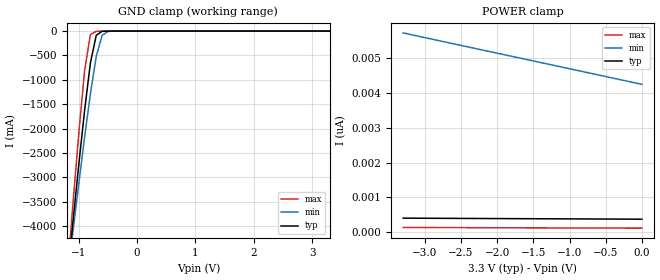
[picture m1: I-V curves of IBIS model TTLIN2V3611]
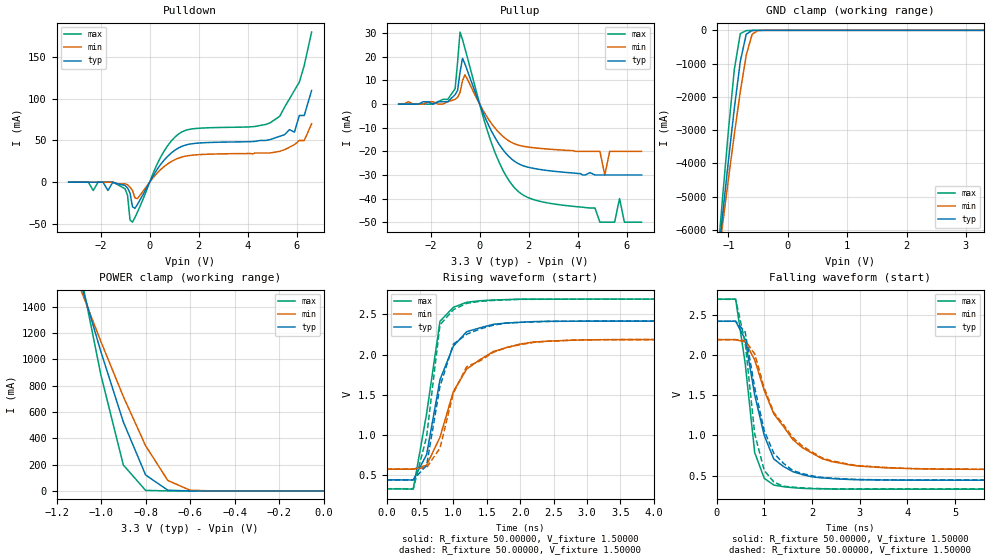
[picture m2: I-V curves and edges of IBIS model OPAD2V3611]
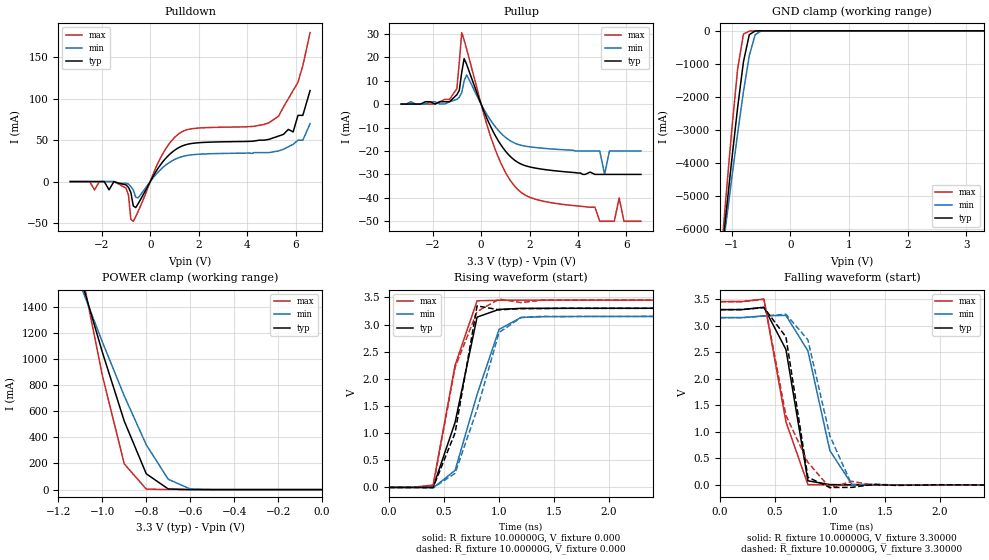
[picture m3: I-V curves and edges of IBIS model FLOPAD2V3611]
| IBIS file 2103pf.ibs created by s2ibis2 version 1.2
| North Carolina State University Electronics Research Laboratory  1995
[IBIS ver]   2.1
[File name]   72v2103p.ibs
[File Rev]   1.0
[Date]   Friday, April 4, 2003
[Source]   IDT
[Notes]   1. Temp typ=25C, min=-40C, max=85C
   2. IDT C11_5_3V_SAC_2M process
   3. Ramp rates based on 50 ohm load
[Disclaimer]
READ THESE TERMS AND CONDITIONS CAREFULLY BEFORE USING THIS IBIS MODEL.  BY
USING THIS IBIS MODEL, YOU ARE ACCEPTING AND AGREEING TO THESE TERMS AND
CONDITIONS OF USE.
Integrated Device Technology, Inc. ("IDT") hereby grants the user of this
IBIS model ("User") a non-exclusive, nontransferable license to use this
IBIS model under the following terms: The User is granted this license only
to use the IBIS model for demonstration purposes only and is not granted
rights to sell, copy (except as needed to run the IBIS model), rent, lease
or sub-license (except for demonstration) the IBIS model in whole or in
part, or in modified form to anyone. The User may modify the IBIS model to
suit its specific applications, but  rights to derivative works and such
modifications shall belong to IDT.
THIS IBIS MODEL IS PROVIDED ON AN AS IS" BASIS AND IDT  MAKES ABSOLUTELY NO
WARRANTY WITH RESPECT TO THE INFORMATION CONTAINED HEREIN.  IDT DISCLAIMS
AND USER WAIVES ALL WARRANTIES, EXPRESS AND IMPLIED, INCLUDING WARRANTIES OF
MERCHANTABILITY AND FITNESS FOR A PARTICULAR PURPOSE.  THE ENTIRE RISK AS TO
QUALITY AND PERFORMANCE IS WITH THE USER  ACCORDINGLY, IN NO EVENT SHALL IDT
BE LIABLE FOR ANY DIRECT OR INDIRECT DAMAGES, WHETHER IN CONTRACT OR TORT,
INCLUDING ANY LOST PROFITS OR OTHER INCIDENTAL, CONSEQUENTIAL, EXEMPLARY, OR
PUNITIVE DAMAGES ARISING OUT OF THE USE OR APPLICATION OF THE  IBIS MODEL,
WHETHER OR NOT IDT HAD NOTICE OF SUCH DAMAGES.
IDT reserves the right to make changes without notice to any product herein
to improve reliability, function, or design. IDT does not convey any license
under patent rights or any other intellectual property rights, including
those of third parties. IDT is not obligated to provide maintenance or
support for the licensed IBIS model.
This model is for the 3.3v High-Density Supersync II 36-Bit FIFO
[Copyright]
Copyright 2002, Integrated Device Technology, Inc. All rights reserved.
|   Component 72V2103PF
[Component]   72V2103PF
[Manufacturer]   Integrated Device Technology Inc.
[Package]
| variable   typ   min   max
R_pkg   0.12500   0.10600   0.15300
L_pkg   6.47000nH   5.60000nH   7.62000nH
C_pkg   0.18200pF   0.16000pF   0.21500pF
[Pin]  signal_name   model_name   R_pin   L_pin   C_pin
1   /WEN   TTLIN2V3611
2   /SEN   TTLIN2V3611
3   NC   NC
4   VCC   POWER
5   NC   NC
6   IW   TTLIN2V3611
7   GND   GND
8   D17   TTLIN2V3611
9   VCC   POWER
10   D16   TTLIN2V3611
11   D15   TTLIN2V3611
12   D14   TTLIN2V3611
13   D13   TTLIN2V3611
14   GND   GND
15   D12   TTLIN2V3611
16   D11   TTLIN2V3611
17   D10   TTLIN2V3611
18   D9   TTLIN2V3611
19   D8   TTLIN2V3611
20   VCC   POWER
21   D7   TTLIN2V3611
22   D6   TTLIN2V3611
23   GND   GND
24   D5   TTLIN2V3611
25   D4   TTLIN2V3611
26   D3   TTLIN2V3611
27   D2   TTLIN2V3611
28   D1   TTLIN2V3611
29   D0   TTLIN2V3611
30   GND   GND
31   Q0   OPAD2V3611
32   Q1   OPAD2V3611
33   GND   GND
34   Q2   OPAD2V3611
35   Q3   OPAD2V3611
36   VCC   POWER
37   Q4   OPAD2V3611
38   Q5   OPAD2V3611
39   GND   GND
40   Q6   OPAD2V3611
41   Q7   OPAD2V3611
42   Q8   OPAD2V3611
43   Q9   OPAD2V3611
44   VCC   POWER
45   Q10   OPAD2V3611
46   GND   GND
47   Q11   OPAD2V3611
48   GND   GND
49   Q12   OPAD2V3611
50   Q13   OPAD2V3611
51   VCC   POWER
52   Q14   OPAD2V3611
53   Q15   OPAD2V3611
54   GND   GND
55   GND   GND
56   Q16   OPAD2V3611
57   Q17   OPAD2V3611
58   VCC   POWER
59   /OE   TTLIN2V3611
60   /RT   TTLIN2V3611
61   /REN   TTLIN2V3611
62   RCLK   TTLIN2V3611
63   RM   TTLIN2V3611
64   /EF-/OR   FLOPAD2V3611
65   PFM   TTLIN2V3611
66   /PAE   FLOPAD2V3611
67   VCC   POWER
68   IP   TTLIN2V3611
69   /BE   TTLIN2V3611
70   FSEL1   TTLIN2V3611
71   /HF   FLOPAD2V3611
72   FSEL0   TTLIN2V3611
73   OW   TTLIN2V3611
74   /PAF   FLOPAD2V3611
75   /FF-/IR   FLOPAD2V3611
76   FWFT/SI   TTLIN2V3611
77   /LD   TTLIN2V3611
78   /MRS   TTLIN2V3611
79   /PRS   TTLIN2V3611
80   WCLK   TTLIN2V3611
|   Model TTLPU2V3611
[Model]   TTLPU2V3611
Model_type   Input
Polarity   Non-Inverting
Vinl =  0.80000V
Vinh =  2.00000V
C_comp   10.00000pF   10.00000pF   10.00000pF
[Temperature Range]   25.00000   85.00000   -40.00000
[Voltage Range]   3.30000V   3.15000V   3.45000V
| End [Model] TTLPU2V3611
| Models and submodels in the file (4): TTLIN2V3611 (Input), TTLPU2V3611 (Input), OPAD2V3611 (3-state), FLOPAD2V3611 (3-state)
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| in   in   dummy_model
| oe   oe   dummy_model
| in1  in1   dummy_model
| oe1  oe1   dummy_model
|   Model TTLIN2V3611
[Model]   TTLIN2V3611
Model_type   Input
Polarity   Non-Inverting
Vinl =  0.80000V
Vinh =  2.00000V
C_comp   10.00000pF   10.00000pF   10.00000pF
[Temperature Range]   25.00000   85.00000   -40.00000
[Voltage Range]   3.30000V   3.15000V   3.45000V
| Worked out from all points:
|   GND clamp passes 1 mA (typ) near -0.51 V on its own axis
[GND_clamp]
| voltage   I(typ)   I(min)   I(max)
-3.3V     -31.62A    -27.14A    -38.3A
-1.2V     -5.12A     -5.123A    -5.052A
-1.1V     -3.918A    -4.12A     -3.553A
-1V       -2.746A    -3.136A    -2.109A
-900mV    -1.631A    -2.183A    -811.7mA
-800mV    -652.4mA   -1.286A    -71.19mA
-700mV    -87.47mA   -520.5mA   -5.646mA
-600mV    -5.364mA   -87.77mA   -1.458mA
-500mV    -302uA     -8.09mA    -219uA
3.3V      373pA      4.31nA     115.1pA
[POWER_clamp]
| voltage   I(typ)   I(min)   I(max)
-3.3V     403.8pA    5.719nA    136.4pA
-2.6V     396.7pA    5.404nA    131.5pA
-1.3V     385pA      4.825nA    123.6pA
0V        373pA      4.243nA    116pA
|   Model OPAD2V3611
[Model]   OPAD2V3611
Model_type   3-state
Polarity   Non-Inverting
Enable   Active-High
Vmeas =  1.50000V
C_comp   10.00000pF   10.00000pF   10.00000pF
[Temperature Range]   25.00000   85.00000   -40.00000
[Voltage Range]   3.30000V   3.15000V   3.45000V
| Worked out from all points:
|   slope of the pulldown table from 0 to 0.495 V, typ, clamps not added: 21.5 ohm
|   slope of the pullup table from 0 to 0.495 V, typ, clamps not added: 42.4 ohm
|   GND clamp passes 1 mA (typ) near -0.52 V on its own axis
|   POWER clamp passes 1 mA (typ) near -0.62 V on its own axis
|   rising waveform, R_fixture 50.00000, V_fixture 1.50000: 20-80 % time 343ps typ, 520ps min, 265ps max; typ from 0.444 V to 2.42 V
|   rising waveform, R_fixture 50.00000, V_fixture 1.50000: 20-80 % time 315ps typ, 424ps min, 232ps max; typ from 0.446 V to 2.42 V
|   falling waveform, R_fixture 50.00000, V_fixture 1.50000: 20-80 % time 461ps typ, 858ps min, 278ps max; typ from 2.42 V to 0.444 V
|   falling waveform, R_fixture 50.00000, V_fixture 1.50000: 20-80 % time 481ps typ, 869ps min, 318ps max; typ from 2.42 V to 0.446 V
[Pulldown]
| voltage   I(typ)   I(min)   I(max)
-3.3V     0A         0A         0A
-1V       -4mA       -2mA       -8mA
-800mV    -13.1mA    -6mA       -45.44mA
-700mV    -29.4mA    -10mA      -47.99mA
-500mV    -26.74mA   -19.63mA   -36.09mA
400mV     19.36mA    13.74mA    27.32mA
1.2V      41.38mA    29.07mA    58.2mA
5.3V      55mA       37mA       79mA
5.9V      60mA       45mA       110mA
6.1V      80mA       50mA       120mA
6.3V      80mA       50mA       140mA
6.6V      110mA      70mA       180mA
[Pullup]
| voltage   I(typ)   I(min)   I(max)
-3.3V     0A         0A         0A
-1.3V     1mA        1mA        2mA
-1V       4mA        2mA        6.5mA
-800mV    13.4mA     4.9mA      30.49mA
-600mV    17.05mA    12.41mA    23.59mA
500mV     -11.77mA   -8.469mA   -17mA
1.5V      -24.75mA   -17.12mA   -36.28mA
4.9V      -30mA      -20mA      -50mA
5.1V      -30mA      -30mA      -50mA
5.7V      -30mA      -20mA      -40mA
5.9V      -30mA      -20mA      -50mA
6.6V      -30mA      -20mA      -50mA
[GND_clamp]
| voltage   I(typ)   I(min)   I(max)
-3.3V     -44.86A    -38.5A     -54.32A
-1.2V     -7.292A    -7.294A    -7.196A
-1.1V     -5.587A    -5.872A    -5.069A
-1V       -3.924A    -4.477A    -3.02A
-900mV    -2.338A    -3.123A    -1.172A
-800mV    -940.2mA   -1.846A    -98.36mA
-700mV    -115.7mA   -749mA     -8.05mA
-600mV    -4.278mA   -114.8mA   -2.238mA
-500mV    -295.2uA   -5.816mA   -325.4uA
3.3V      607.7pA    5.602nA    92.71pA
[POWER_clamp]
| voltage   I(typ)   I(min)   I(max)
-3.3V     15.46A     11.9A      22.55A
-1.1V     1.627A     1.567A     1.714A
-1V       1.053A     1.131A     875.2mA
-900mV    523.9mA    716.9mA    196.8mA
-800mV    121.2mA    343.1mA    4.086mA
-700mV    5.031mA    78.95mA    112.4uA
-600mV    111.5uA    5.081mA    8.814uA
0V        607.7pA    2.814nA    110.2pA
[Ramp]
| variable   typ   min   max
dV/dt_r   0.80040/0.49852n   0.55518/0.74186n   1.11420/0.33285n
dV/dt_f   1.24980/0.73875n   0.95160/1.28926n   1.51836/0.39958n
R_load = 50.00000
[Rising Waveform]
R_fixture = 50.00000
V_fixture = 1.50000
V_fixture_min = 1.50000
V_fixture_max = 1.50000
| time   V(typ)   V(min)   V(max)
0s        444.1mV    577.5mV    332.7mV
400ps     443.2mV    577.5mV    329.4mV
600ps     759mV      626.9mV    1.268V
800ps     1.69V      974.8mV    2.415V
1ns       2.105V     1.542V     2.588V
1.2ns     2.286V     1.821V     2.651V
1.6ns     2.377V     2.039V     2.679V
2ns       2.402V     2.131V     2.689V
2.4ns     2.414V     2.167V     2.69V
10ns      2.417V     2.189V     2.691V
[Rising Waveform]
R_fixture = 50.00000
V_fixture = 1.50000
V_fixture_min = 1.50000
V_fixture_max = 1.50000
R_dut = 0.12500
L_dut = 6.47000nH
C_dut = 0.18200pF
| time   V(typ)   V(min)   V(max)
0s        445.9mV    578.8mV    334.9mV
400ps     445.7mV    578.8mV    334.3mV
600ps     624.2mV    598mV      981.7mV
800ps     1.607V     838.6mV    2.371V
1ns       2.13V      1.522V     2.559V
1.2ns     2.254V     1.851V     2.638V
1.6ns     2.367V     2.03V      2.675V
1.8ns     2.394V     2.091V     2.682V
2.4ns     2.413V     2.166V     2.688V
10ns      2.416V     2.188V     2.689V
[Falling Waveform]
R_fixture = 50.00000
V_fixture = 1.50000
V_fixture_min = 1.50000
V_fixture_max = 1.50000
| time   V(typ)   V(min)   V(max)
0s        2.417V     2.189V     2.691V
400ps     2.417V     2.189V     2.692V
600ps     2.192V     2.159V     1.896V
800ps     1.502V     1.937V     786.7mV
1ns       1V         1.557V     467.2mV
1.2ns     707.2mV    1.267V     383.9mV
1.8ns     513.6mV    846.8mV    342.6mV
2.2ns     473.3mV    714.4mV    336.7mV
2.8ns     452.6mV    633mV      333.3mV
10ns      444.1mV    577.6mV    332.7mV
[Falling Waveform]
R_fixture = 50.00000
V_fixture = 1.50000
V_fixture_min = 1.50000
V_fixture_max = 1.50000
R_dut = 0.12500
L_dut = 6.47000nH
C_dut = 0.18200pF
| time   V(typ)   V(min)   V(max)
0s        2.416V     2.188V     2.689V
400ps     2.417V     2.188V     2.689V
600ps     2.283V     2.175V     2.153V
800ps     1.591V     2.01V      1.017V
1ns       1.059V     1.589V     565mV
1.2ns     778.4mV    1.284V     421.6mV
1.4ns     654.9mV    1.135V     368.5mV
2.2ns     479.3mV    723.9mV    339.7mV
3ns       452.9mV    622.8mV    335.3mV
10ns      445.9mV    578.8mV    334.9mV
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|   Model FLOPAD2V3611
[Model]   FLOPAD2V3611
Model_type   3-state
Polarity   Non-Inverting
Enable   Active-High
Vmeas =  1.50000V
C_comp   10.00000pF   10.00000pF   10.00000pF
[Temperature Range]   25.00000   85.00000   -40.00000
[Voltage Range]   3.30000V   3.15000V   3.45000V
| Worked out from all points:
|   slope of the pulldown table from 0 to 0.495 V, typ, clamps not added: 21.5 ohm
|   slope of the pullup table from 0 to 0.495 V, typ, clamps not added: 42.4 ohm
|   GND clamp passes 1 mA (typ) near -0.52 V on its own axis
|   POWER clamp passes 1 mA (typ) near -0.62 V on its own axis
|   rising waveform, R_fixture 10.00000G, V_fixture 0.000: 20-80 % time 239ps typ, 290ps min, 227ps max; typ from 0 V to 3.3 V
|   rising waveform, R_fixture 10.00000G, V_fixture 0.000: 20-80 % time 208ps typ, 290ps min, 247ps max; typ from 0 V to 3.3 V
|   falling waveform, R_fixture 10.00000G, V_fixture 3.30000: 20-80 % time 175ps typ, 205ps min, 221ps max; typ from 3.3 V to 0 V
|   falling waveform, R_fixture 10.00000G, V_fixture 3.30000: 20-80 % time 150ps typ, 241ps min, 273ps max; typ from 3.3 V to -0.001 V
[Pulldown]
| voltage   I(typ)   I(min)   I(max)
-3.3V     0A         0A         0A
-1V       -4mA       -2mA       -8mA
-800mV    -13.1mA    -6mA       -45.44mA
-700mV    -29.4mA    -10mA      -47.99mA
-500mV    -26.74mA   -19.63mA   -36.09mA
400mV     19.36mA    13.74mA    27.32mA
1.2V      41.38mA    29.07mA    58.2mA
5.3V      55mA       37mA       79mA
5.9V      60mA       45mA       110mA
6.1V      80mA       50mA       120mA
6.3V      80mA       50mA       140mA
6.6V      110mA      70mA       180mA
[Pullup]
| voltage   I(typ)   I(min)   I(max)
-3.3V     0A         0A         0A
-1.3V     1mA        1mA        2mA
-1V       4mA        2mA        6.6mA
-800mV    13.4mA     4.9mA      30.49mA
-600mV    17.05mA    12.41mA    23.59mA
500mV     -11.77mA   -8.469mA   -17mA
1.5V      -24.75mA   -17.12mA   -36.28mA
4.9V      -30mA      -20mA      -50mA
5.1V      -30mA      -30mA      -50mA
5.7V      -30mA      -20mA      -40mA
5.9V      -30mA      -20mA      -50mA
6.6V      -30mA      -20mA      -50mA
[GND_clamp]
| voltage   I(typ)   I(min)   I(max)
-3.3V     -44.86A    -38.5A     -54.32A
-1.2V     -7.292A    -7.294A    -7.196A
-1.1V     -5.587A    -5.872A    -5.069A
-1V       -3.924A    -4.477A    -3.02A
-900mV    -2.338A    -3.123A    -1.172A
-800mV    -940.2mA   -1.846A    -98.36mA
-700mV    -115.7mA   -749mA     -8.05mA
-600mV    -4.278mA   -114.8mA   -2.238mA
-500mV    -295.2uA   -5.816mA   -325.4uA
3.3V      607.7pA    5.602nA    92.72pA
[POWER_clamp]
| voltage   I(typ)   I(min)   I(max)
-3.3V     15.46A     11.9A      22.55A
-1.1V     1.627A     1.567A     1.714A
-1V       1.053A     1.131A     875.2mA
-900mV    523.9mA    716.9mA    196.8mA
-800mV    121.2mA    343.1mA    4.086mA
-700mV    5.031mA    78.95mA    112.4uA
-600mV    111.5uA    5.081mA    8.814uA
0V        607.7pA    2.814nA    110.2pA
[Ramp]
| variable   typ   min   max
dV/dt_r   0.80040/0.24935n   0.55518/0.34835n   1.11420/0.17021n
dV/dt_f   1.24980/0.48363n   0.95160/0.80240n   1.51836/0.26104n
R_load = 50.00000
[Rising Waveform]
R_fixture = 10.00000G
V_fixture = 0.000
V_fixture_min = 0.000
V_fixture_max = 0.000
| time   V(typ)   V(min)   V(max)
0s        0V         0V         0V
200ps     -592.5uV   -37.45uV   -1.019mV
400ps     3.601mV    -8.441mV   43.48mV
600ps     1.197V     314.4mV    2.251V
800ps     3.137V     1.711V     3.438V
1ns       3.28V      2.91V      3.448V
1.2ns     3.298V     3.131V     3.449V
1.8ns     3.299V     3.149V     3.45V
10ns      3.3V       3.15V      3.45V
[Rising Waveform]
R_fixture = 10.00000G
V_fixture = 0.000
V_fixture_min = 0.000
V_fixture_max = 0.000
R_dut = 0.12500
L_dut = 6.47000nH
C_dut = 0.18200pF
| time   V(typ)   V(min)   V(max)
0s        0V         0V         0V
200ps     -218.2uV   296uV      -616.5uV
400ps     -2.633mV   -8.312mV   24.23mV
600ps     1.006V     260.1mV    2.212V
800ps     3.344V     1.434V     3.238V
1ns       3.271V     2.853V     3.468V
1.2ns     3.294V     3.129V     3.405V
1.4ns     3.295V     3.151V     3.45V
10ns      3.3V       3.15V      3.455V
[Falling Waveform]
R_fixture = 10.00000G
V_fixture = 3.30000
V_fixture_min = 3.15000
V_fixture_max = 3.45000
| time   V(typ)   V(min)   V(max)
0s        3.3V       3.15V      3.45V
200ps     3.301V     3.15V      3.453V
400ps     3.345V     3.183V     3.498V
600ps     2.552V     3.192V     1.191V
800ps     79.6mV     2.525V     8.023mV
1ns       8.737mV    647.8mV    3.594mV
1.2ns     4.579mV    12.73mV    1.742mV
10ns      2.865uV    0V         3.049uV
[Falling Waveform]
R_fixture = 10.00000G
V_fixture = 3.30000
V_fixture_min = 3.15000
V_fixture_max = 3.45000
R_dut = 0.12500
L_dut = 6.47000nH
C_dut = 0.18200pF
| time   V(typ)   V(min)   V(max)
0s        3.3V       3.15V      3.45V
200ps     3.3V       3.149V     3.451V
400ps     3.338V     3.179V     3.494V
600ps     2.787V     3.214V     1.312V
800ps     146.2mV    2.731V     426.9mV
1ns       -45.77mV   925.3mV    -52.66mV
1.2ns     -43.3mV    1.552mV    69.38mV
1.4ns     13.04mV    16.7mV     -1.508mV
1.6ns     -6.432mV   -261.5uV   184.5uV
10ns      -737.5uV   109.8uV    75.85uV
